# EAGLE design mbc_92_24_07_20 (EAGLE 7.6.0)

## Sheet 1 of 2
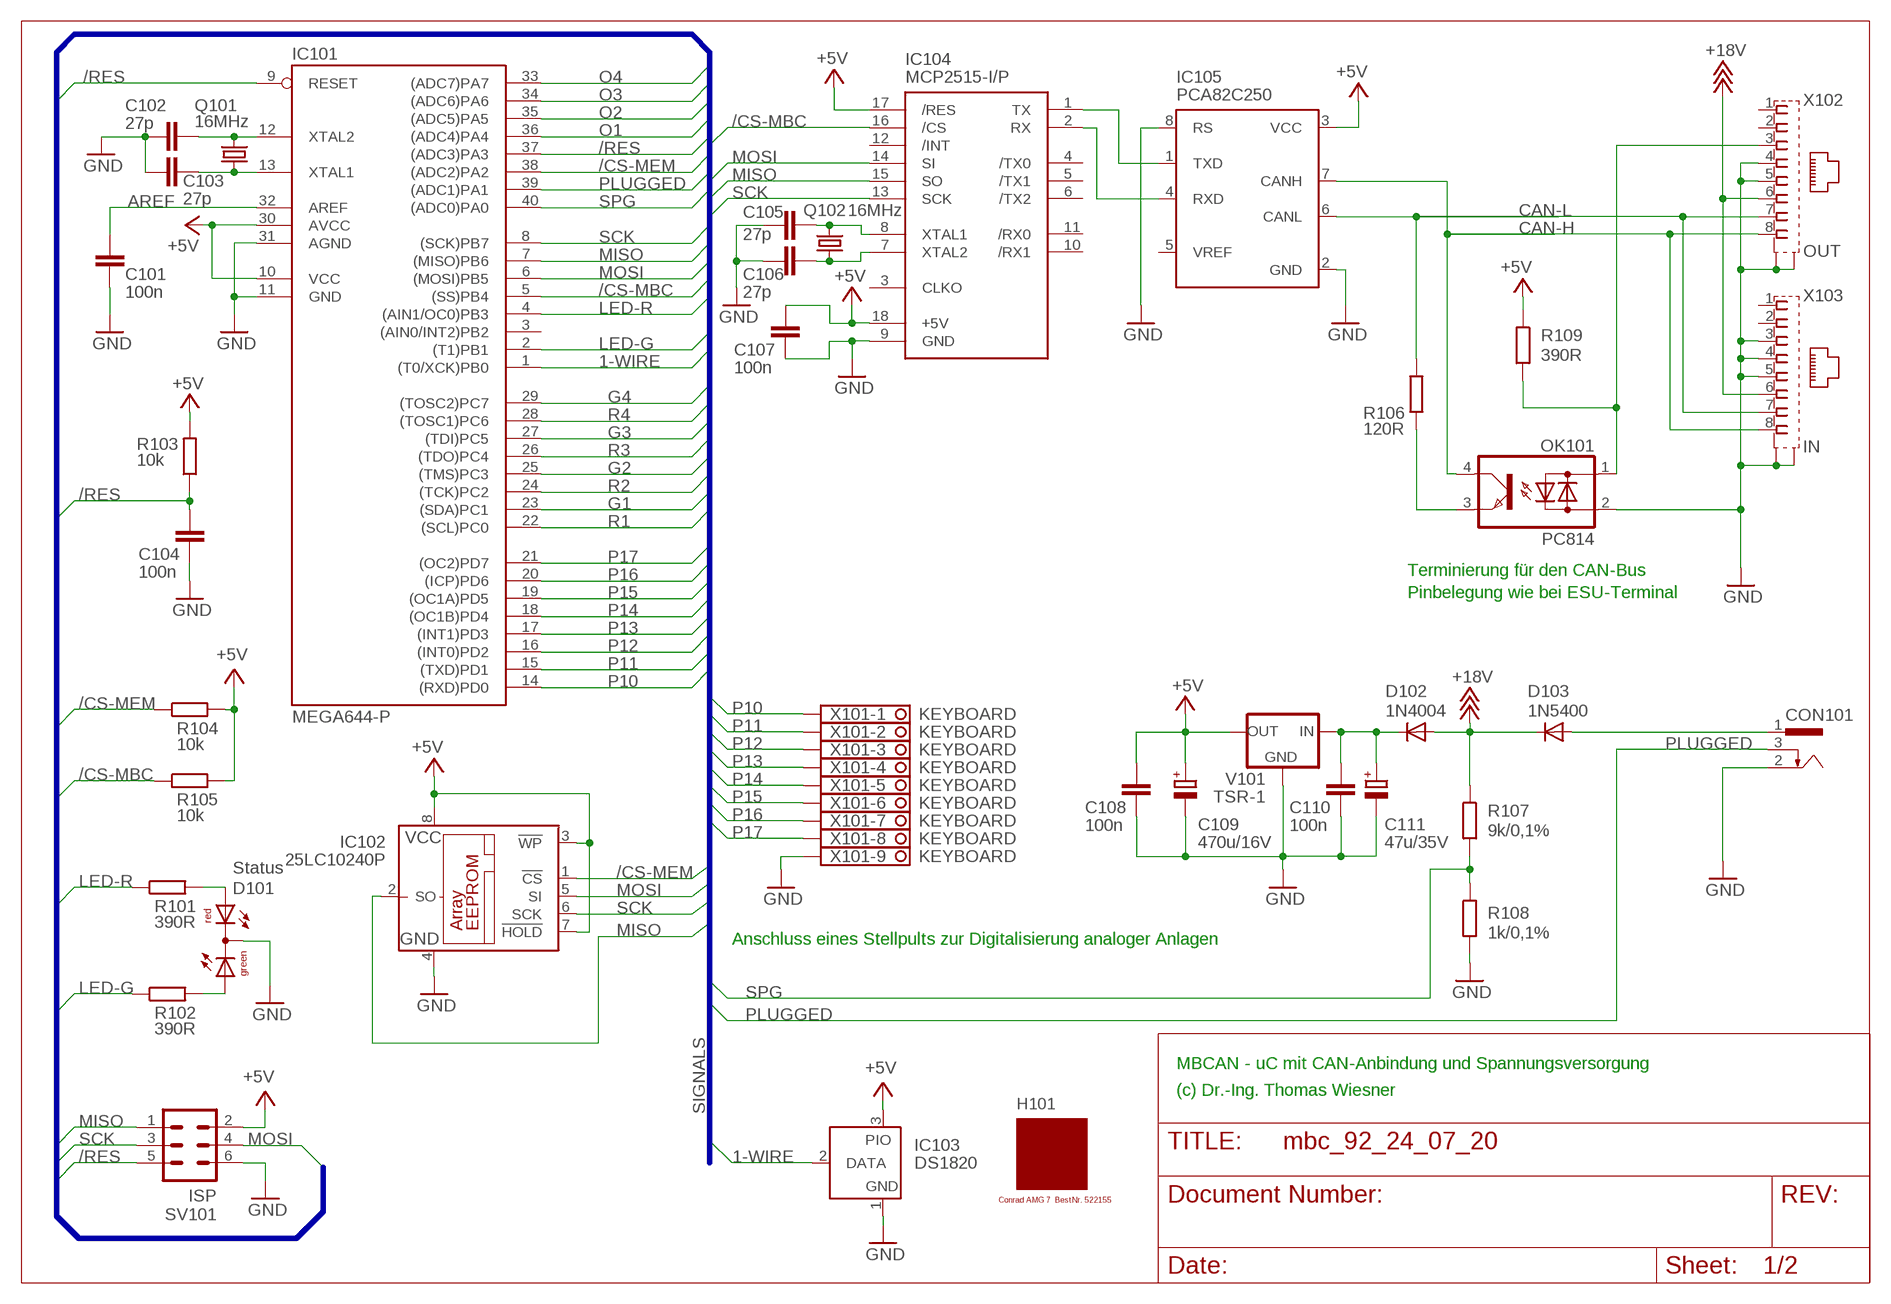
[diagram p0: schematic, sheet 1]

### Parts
C101  100n  C-EU025-025X050  [C025-025X050]
C102  27p  C-EU025-025X050  [C025-025X050]
C103  27p  C-EU025-025X050  [C025-025X050]
C104  100n  C-EU025-025X050  [C025-025X050]
C105  27p  C-EU025-025X050  [C025-025X050]
C106  27p  C-EU025-025X050  [C025-025X050]
C107  100n  C-EU025-025X050  [C025-025X050]
C108  100n  C-EU025-025X050  [C025-025X050]
C109  470u/16V  CPOL-EUE3.5-8  [E3,5-8]
C110  100n  C-EU025-025X050  [C025-025X050]
C111  47u/35V  CPOL-EUE2.5-7  [E2,5-7]
CON101  POWER-JACK  [POWER-JACK]
D101  Status  DUOLED5MM  [DUOLED5MM]
D102  1N4004  [DO41-10]
D103  1N5400  [DO201-15]
H101  MODULGEHÄUSE-AMG-7  [MODULGEHÄUSE-1]
IC101  MEGA644-P  MEGA323-P  [DIL40]
IC102  25LC10240P  25LC040P  [DIL8]
IC103  DS1820  DS2405  [TO92-]
IC104  MCP2515-I/P  MCP2510-I/P  [DIL18]
IC105  PCA82C250  [DIL08]
OK101  PC814  [DIL04]
Q101  16MHz  CRYSTALHC49U70  [HC49U70]
Q102  16MHz  CRYSTALHC49U70  [HC49U70]
R101  390R  R-EU_0207/10  [0207/10]
R102  390R  R-EU_0207/10  [0207/10]
R103  10k  R-EU_0207/10  [0207/10]
R104  10k  R-EU_0207/10  [0207/10]
R105  10k  R-EU_0207/10  [0207/10]
R106  120R  R-EU_0207/10  [0207/10]
R107  9k/0,1%  R-EU_0207/10  [0207/10]
R108  1k/0,1%  R-EU_0207/10  [0207/10]
R109  390R  R-EU_0207/10  [0207/10]
SV101  ISP  ML6  [ML6]
V101  TSR-1  [TRACO-TSR-1]
X101  KEYBOARD  1751316  [1751316]
X102  OUT  0446200002  [0446200002]
X103  IN  0446200002  [0446200002]

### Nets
1-WIRE: IC101.1((T0/XCK)PB0) IC103.2(DATA)
+5V: C107.1 C108.1 C109.+ IC101.10(VCC) IC101.30(AVCC) IC102.3(!WP) IC102.7(!HOLD) IC102.8(VCC) IC103.3(PIO) IC104.17(/RES) IC104.18(+5V) IC105.3(VCC) R103.2 R104.2 R105.2 R109.1 SV101.2 V101.OUT ; also sheet 2
+18V: D102.A D103.C R107.1 X102.6 X103.6
/CS-MBC: IC101.5((SS)PB4) IC104.16(/CS) R105.1
/CS-MEM: IC101.38((ADC2)PA2) IC102.1(!CS) R104.1
/RES: C104.1 IC101.9(RESET) IC101.37((ADC3)PA3) R103.1 SV101.5
AREF: C101.1 IC101.32(AREF)
CAN-H: IC105.7(CANH) OK101.4(C) X102.8 X103.8
CAN-L: IC105.6(CANL) R106.2 X102.7 X103.7
G1: IC101.23((SDA)PC1) ; also sheet 2
G2: IC101.25((TMS)PC3) ; also sheet 2
G3: IC101.27((TDI)PC5) ; also sheet 2
G4: IC101.29((TOSC2)PC7) ; also sheet 2
GND: C101.2 C102.1 C103.1 C104.2 C105.1 C106.1 C107.2 C108.2 C109.- C110.2 C111.- CON101.2 D101.K(C) IC101.11(GND) IC101.31(AGND) IC102.4(GND) IC103.1(GND) IC104.9(GND) IC105.2(GND) IC105.8(RS) OK101.2(AC2) R108.2 SV101.6 V101.GND X101.9 X102.4 X102.5 X102.S@1(S1) X102.S@2(S2) X103.3 X103.4 X103.5 X103.S@1(S1) X103.S@2(S2) ; also sheet 2
LED-G: IC101.2((T1)PB1) R102.1
LED-R: IC101.4((AIN1/OC0)PB3) R101.1
MISO: IC101.7((MISO)PB6) IC102.2(SO) IC104.15(SO) SV101.1
MOSI: IC101.6((MOSI)PB5) IC102.5(SI) IC104.14(SI) SV101.4
N$1: IC104.1(TX) IC105.1(TXD)
N$2: IC104.2(RX) IC105.4(RXD)
N$3: OK101.3(E) R106.1
N$4: OK101.1(AC1) R109.2 X102.3
N$6: C110.1 C111.+ D102.C V101.IN
N$9: D101.AR R101.2
N$13: D101.AG R102.2
N$40: C102.2 IC101.12(XTAL2) Q101.2
N$41: C103.2 IC101.13(XTAL1) Q101.1
N$42: C105.2 IC104.8(XTAL1) Q102.2
N$43: C106.2 IC104.7(XTAL2) Q102.1
O1: IC101.36((ADC4)PA4) ; also sheet 2
O2: IC101.35((ADC5)PA5) ; also sheet 2
O3: IC101.34((ADC6)PA6) ; also sheet 2
O4: IC101.33((ADC7)PA7) ; also sheet 2
P10: IC101.14((RXD)PD0) X101.1
P11: IC101.15((TXD)PD1) X101.2
P12: IC101.16((INT0)PD2) X101.3
P13: IC101.17((INT1)PD3) X101.4
P14: IC101.18((OC1B)PD4) X101.5
P15: IC101.19((OC1A)PD5) X101.6
P16: IC101.20((ICP)PD6) X101.7
P17: IC101.21((OC2)PD7) X101.8
PLUGGED: CON101.3 IC101.39((ADC1)PA1)
R1: IC101.22((SCL)PC0) ; also sheet 2
R2: IC101.24((TCK)PC2) ; also sheet 2
R3: IC101.26((TDO)PC4) ; also sheet 2
R4: IC101.28((TOSC1)PC6) ; also sheet 2
SCK: IC101.8((SCK)PB7) IC102.6(SCK) IC104.13(SCK) SV101.3
SPG: IC101.40((ADC0)PA0) R107.2 R108.1
V-NETZTEIL1: CON101.1 D103.A
Unconnected: IC101.3((AIN0/INT2)PB2) IC104.3(CLKO) IC104.4(/TX0) IC104.5(/TX1) IC104.6(/TX2) IC104.10(/RX1) IC104.11(/RX0) IC104.12(/INT) IC105.5(VREF) X102.1 X102.2 X103.1 X103.2

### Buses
SIGNALS

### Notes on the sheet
- Terminierung für den CAN-Bus
- Pinbelegung wie bei ESU-Terminal
- Anschluss eines Stellpults zur Digitalisierung analoger Anlagen
- MBCAN - uC mit CAN-Anbindung und Spannungsversorgung
- (c) Dr.-Ing. Thomas Wiesner

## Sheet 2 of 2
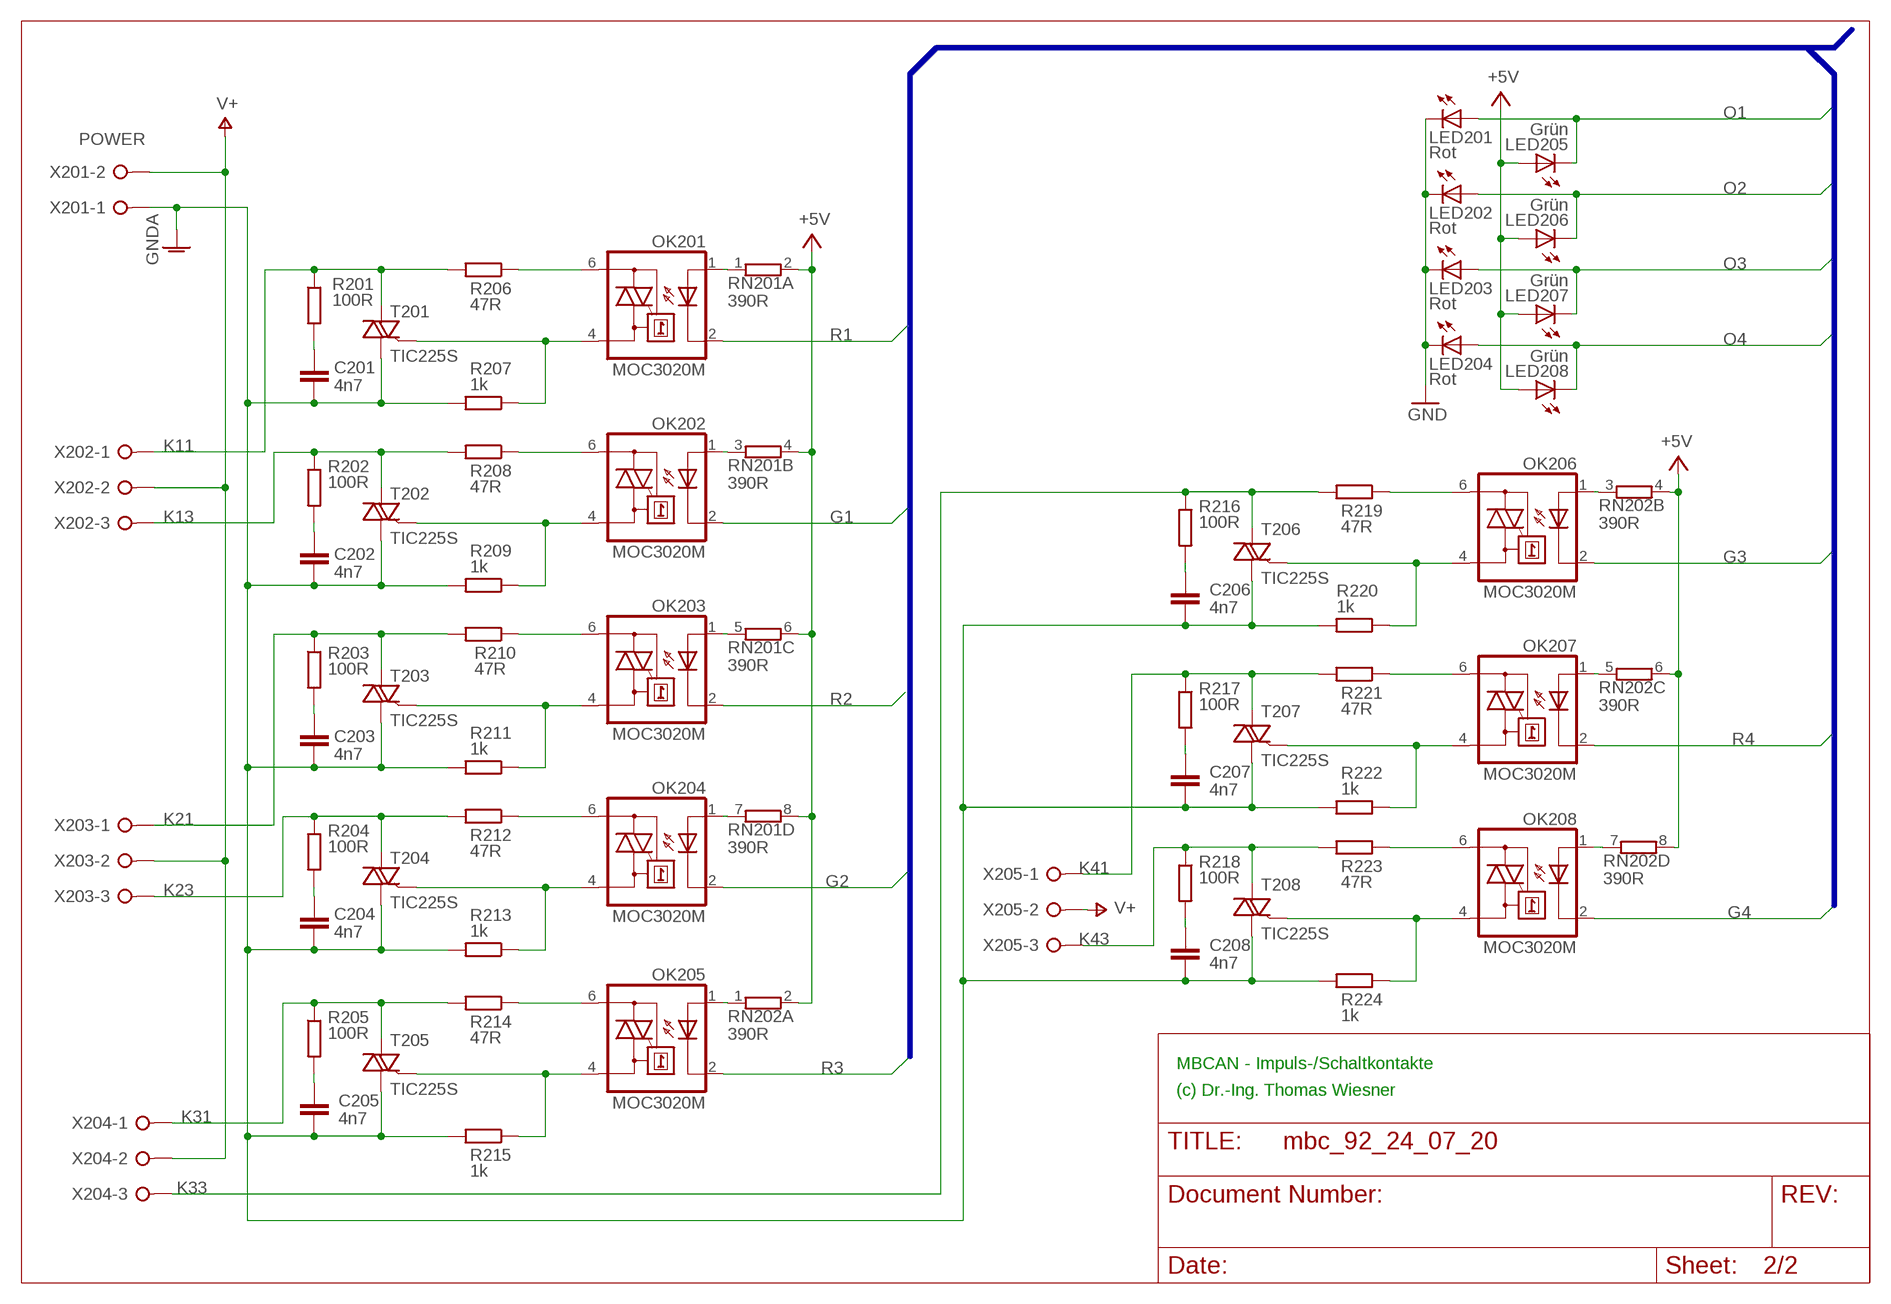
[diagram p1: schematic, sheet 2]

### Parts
C201  4n7  C-EU025-025X050  [C025-025X050]
C202  4n7  C-EU025-025X050  [C025-025X050]
C203  4n7  C-EU025-025X050  [C025-025X050]
C204  4n7  C-EU025-025X050  [C025-025X050]
C205  4n7  C-EU025-025X050  [C025-025X050]
C206  4n7  C-EU025-025X050  [C025-025X050]
C207  4n7  C-EU025-025X050  [C025-025X050]
C208  4n7  C-EU025-025X050  [C025-025X050]
LED201  Rot  LED3MM  [LED3MM]
LED202  Rot  LED3MM  [LED3MM]
LED203  Rot  LED3MM  [LED3MM]
LED204  Rot  LED3MM  [LED3MM]
LED205  Grün  LED3MM  [LED3MM]
LED206  Grün  LED3MM  [LED3MM]
LED207  Grün  LED3MM  [LED3MM]
LED208  Grün  LED3MM  [LED3MM]
OK201  MOC3020M  [DIL06]
OK202  MOC3020M  [DIL06]
OK203  MOC3020M  [DIL06]
OK204  MOC3020M  [DIL06]
OK205  MOC3020M  [DIL06]
OK206  MOC3020M  [DIL06]
OK207  MOC3020M  [DIL06]
OK208  MOC3020M  [DIL06]
R201  100R  R-EU_0207/10  [0207/10]
R202  100R  R-EU_0207/10  [0207/10]
R203  100R  R-EU_0207/10  [0207/10]
R204  100R  R-EU_0207/10  [0207/10]
R205  100R  R-EU_0207/10  [0207/10]
R206  47R  R-EU_0207/10  [0207/10]
R207  1k  R-EU_0207/10  [0207/10]
R208  47R  R-EU_0207/10  [0207/10]
R209  1k  R-EU_0207/10  [0207/10]
R210  47R  R-EU_0207/10  [0207/10]
R211  1k  R-EU_0207/10  [0207/10]
R212  47R  R-EU_0207/10  [0207/10]
R213  1k  R-EU_0207/10  [0207/10]
R214  47R  R-EU_0207/10  [0207/10]
R215  1k  R-EU_0207/10  [0207/10]
R216  100R  R-EU_0207/10  [0207/10]
R217  100R  R-EU_0207/10  [0207/10]
R218  100R  R-EU_0207/10  [0207/10]
R219  47R  R-EU_0207/10  [0207/10]
R220  1k  R-EU_0207/10  [0207/10]
R221  47R  R-EU_0207/10  [0207/10]
R222  1k  R-EU_0207/10  [0207/10]
R223  47R  R-EU_0207/10  [0207/10]
R224  1k  R-EU_0207/10  [0207/10]
RN201  390R  E4R  [SIL8]
RN202  390R  E4R  [SIL8]
T201  TIC225S  [TO220DS]
T202  TIC225S  [TO220DS]
T203  TIC225S  [TO220DS]
T204  TIC225S  [TO220DS]
T205  TIC225S  [TO220DS]
T206  TIC225S  [TO220DS]
T207  TIC225S  [TO220DS]
T208  TIC225S  [TO220DS]
X201  POWER  W237-02P  [W237-132]
X202  W237-03P  [W237-133]
X203  W237-03P  [W237-133]
X204  W237-03P  [W237-133]
X205  W237-03P  [W237-133]

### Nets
+5V: LED205.A LED206.A LED207.A LED208.A RN201.2 RN201.4 RN201.6 RN201.8 RN202.2 RN202.4 RN202.6 RN202.8 ; also sheet 1
G1: OK202.2(C) ; also sheet 1
G2: OK204.2(C) ; also sheet 1
G3: OK206.2(C) ; also sheet 1
G4: OK208.2(C) ; also sheet 1
GND: LED201.K(C) LED202.K(C) LED203.K(C) LED204.K(C) ; also sheet 1
GNDA: C201.2 C202.2 C203.2 C204.2 C205.2 C206.2 C207.2 C208.2 R207.2 R209.2 R211.2 R213.2 R215.2 R220.2 R222.2 R224.2 T201.A1 T202.A1 T203.A1 T204.A1 T205.A1 T206.A1 T207.A1 T208.A1 X201.1
K11: R201.1 R206.2 T201.A2 X202.1
K13: R202.1 R208.2 T202.A2 X202.3
K21: R203.1 R210.2 T203.A2 X203.1
K23: R204.1 R212.2 T204.A2 X203.3
K31: R205.1 R214.2 T205.A2 X204.1
K33: R216.1 R219.2 T206.A2 X204.3
K41: R217.1 R221.2 T207.A2 X205.1
K43: R218.1 R223.2 T208.A2 X205.3
N$5: OK206.1(A) RN202.3
N$7: OK201.1(A) RN201.1
N$8: OK206.4(A1) R220.1 T206.G
N$10: OK201.4(A1) R207.1 T201.G
N$11: OK201.6(A2) R206.1
N$12: OK202.1(A) RN201.3
N$14: OK206.6(A2) R219.1
N$15: C201.1 R201.2
N$16: C206.1 R216.2
N$17: OK202.4(A1) R209.1 T202.G
N$18: OK202.6(A2) R208.1
N$19: OK207.1(A) RN202.5
N$20: C202.1 R202.2
N$21: OK203.1(A) RN201.5
N$22: OK207.4(A1) R222.1 T207.G
N$23: OK203.4(A1) R211.1 T203.G
N$24: OK203.6(A2) R210.1
N$25: OK207.6(A2) R221.1
N$26: C203.1 R203.2
N$27: OK204.1(A) RN201.7
N$28: C207.1 R217.2
N$29: OK204.4(A1) R213.1 T204.G
N$30: OK204.6(A2) R212.1
N$31: OK208.1(A) RN202.7
N$32: C204.1 R204.2
N$33: OK205.1(A) RN202.1
N$34: OK208.4(A1) R224.1 T208.G
N$35: OK205.4(A1) R215.1 T205.G
N$36: OK205.6(A2) R214.1
N$37: OK208.6(A2) R223.1
N$38: C205.1 R205.2
N$39: C208.1 R218.2
O1: LED201.A LED205.K(C) ; also sheet 1
O2: LED202.A LED206.K(C) ; also sheet 1
O3: LED203.A LED207.K(C) ; also sheet 1
O4: LED204.A LED208.K(C) ; also sheet 1
R1: OK201.2(C) ; also sheet 1
R2: OK203.2(C) ; also sheet 1
R3: OK205.2(C) ; also sheet 1
R4: OK207.2(C) ; also sheet 1
V+: X201.2 X202.2 X203.2 X204.2 X205.2

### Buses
B$1

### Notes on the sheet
- MBCAN - Impuls-/Schaltkontakte
- (c) Dr.-Ing. Thomas Wiesner

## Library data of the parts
C101-C108 C110 = rcl:C-EU: CAPACITOR, European symbol
C109 C111 = rcl:CPOL-EU: POLARIZED CAPACITOR, European symbol
C201-C208 = resistor:C-EU: CAPACITOR, European symbol
CON101 = mbc:POWER-JACK: Power-Stecker für 2,5 mm Hohlbuchse
D101 = led:DUOLED5MM: DUO LED 2 colors, 5 mm, round
D102 = diode:1N4004: DIODE
D103 = diode:1N5400: DIODE
H101 = mbc:MODULGEHÄUSE-AMG-7: Gehäuse
IC101 = atmel:MEGA323-P: MICROCONTROLLER 32 Kbytes FLASH 2 Kbytes SRAM 1 Kbytes EEPROM USART 8-channel 10 bit ADC Source: avr.lbr; OC_FARNELL: unknown; OC_NEWARK: unknown
IC102 = microchip:25*: Serial EEPROM 4K/ 8K , SPI bus; MF: MICROCHIP; MPN: 25LC040/P; OC_FARNELL: 9758100; OC_NEWARK: 96K4091
IC103 = maxim:DS2405: Addressable Switch DALLAS Semiconductor; MF: DALLAS SEMICONDUCTOR; MPN: DS2405; OC_FARNELL: 1188025; OC_NEWARK: 06F4645
IC104 = mbc:MCP2510: BASIC-CAN 2.0a Controller Stand-alone CAN controller von Microchip
IC105 = micro-philips:PCA82C250: CAN CONTROLLER INTERFACE; OC_FARNELL: 3692358; OC_NEWARK: unknown
LED201-LED208 = led:LED: LED
OK101 = optocoupler:PC814: SHARP OPTO COUPLER; OC_FARNELL: 9707662; OC_NEWARK: unknown
OK201-OK208 = optocoupler:MOC30*M: RANDOM-PHASE OPTOISOLATORS TRIAC DRIVER OUTPUT Source: http://www.fairchildsemi.com MOC3020-M.pdf; MF: FAIRCHILD SEMICONDUCTOR; MPN: MOC3020-M; OC_FARNELL: 1505425; OC_NEWARK: 72K8895
Q101 Q102 = crystal:CRYSTAL: CRYSTAL; OC_FARNELL: unknown; OC_NEWARK: unknown
R101-R109 R201-R224 = resistor:R-EU_: RESISTOR, European symbol
RN201 RN202 = resistor-sil:E4R: SIL RESISTOR; OC_FARNELL: unknown; OC_NEWARK: unknown
SV101 = con-ml:ML6: HARTING; OC_FARNELL: unknown; OC_NEWARK: unknown
T201-T208 = triac:TIC225S: TRIAC
V101 = mbc:TSR-1: Spannungsregler Hersteller: TRACO Typ: TSR-1 5V: TSR 1-2450 Spg: 5V Strom: 1A Reichelt TSR 1-2450
X101 = con-phoenix-350:1751316: MKDS 1/ 9-3,5 Printklemme Nennstrom: 10 A Bemessungsspannung: 160 V Raster: 3,5 mm Polzahl: 9 Montageart: Löten Anschlussart: Schraubanschluss Anschlussrichtung vom Leiter zur Platine: 0° Source: http://eshop.phoenixcontact.com .. 1751316.pdf; OC_FARNELL: unknown; OC_NEWARK: unknown
X102 X103 = mbc:0446200002: RJ-45 INVERTED MODULAR JACK ASSEMBLY WITH RJ-11 KEEPOUT FEATURE Source: Data sheet MOLEX 0446200002 BUCHSE, RJ45, GESCHIRMT Source: Farnell; MF: MOLEX; MPN: 0446200002; OC_FARNELL: 9251910
X201 = con-wago-508:W237-02P: WAGO SREW CLAMP; OC_FARNELL: unknown; OC_NEWARK: unknown
X202-X205 = con-wago-508:W237-03P: WAGO SREW CLAMP; OC_FARNELL: unknown; OC_NEWARK: unknown

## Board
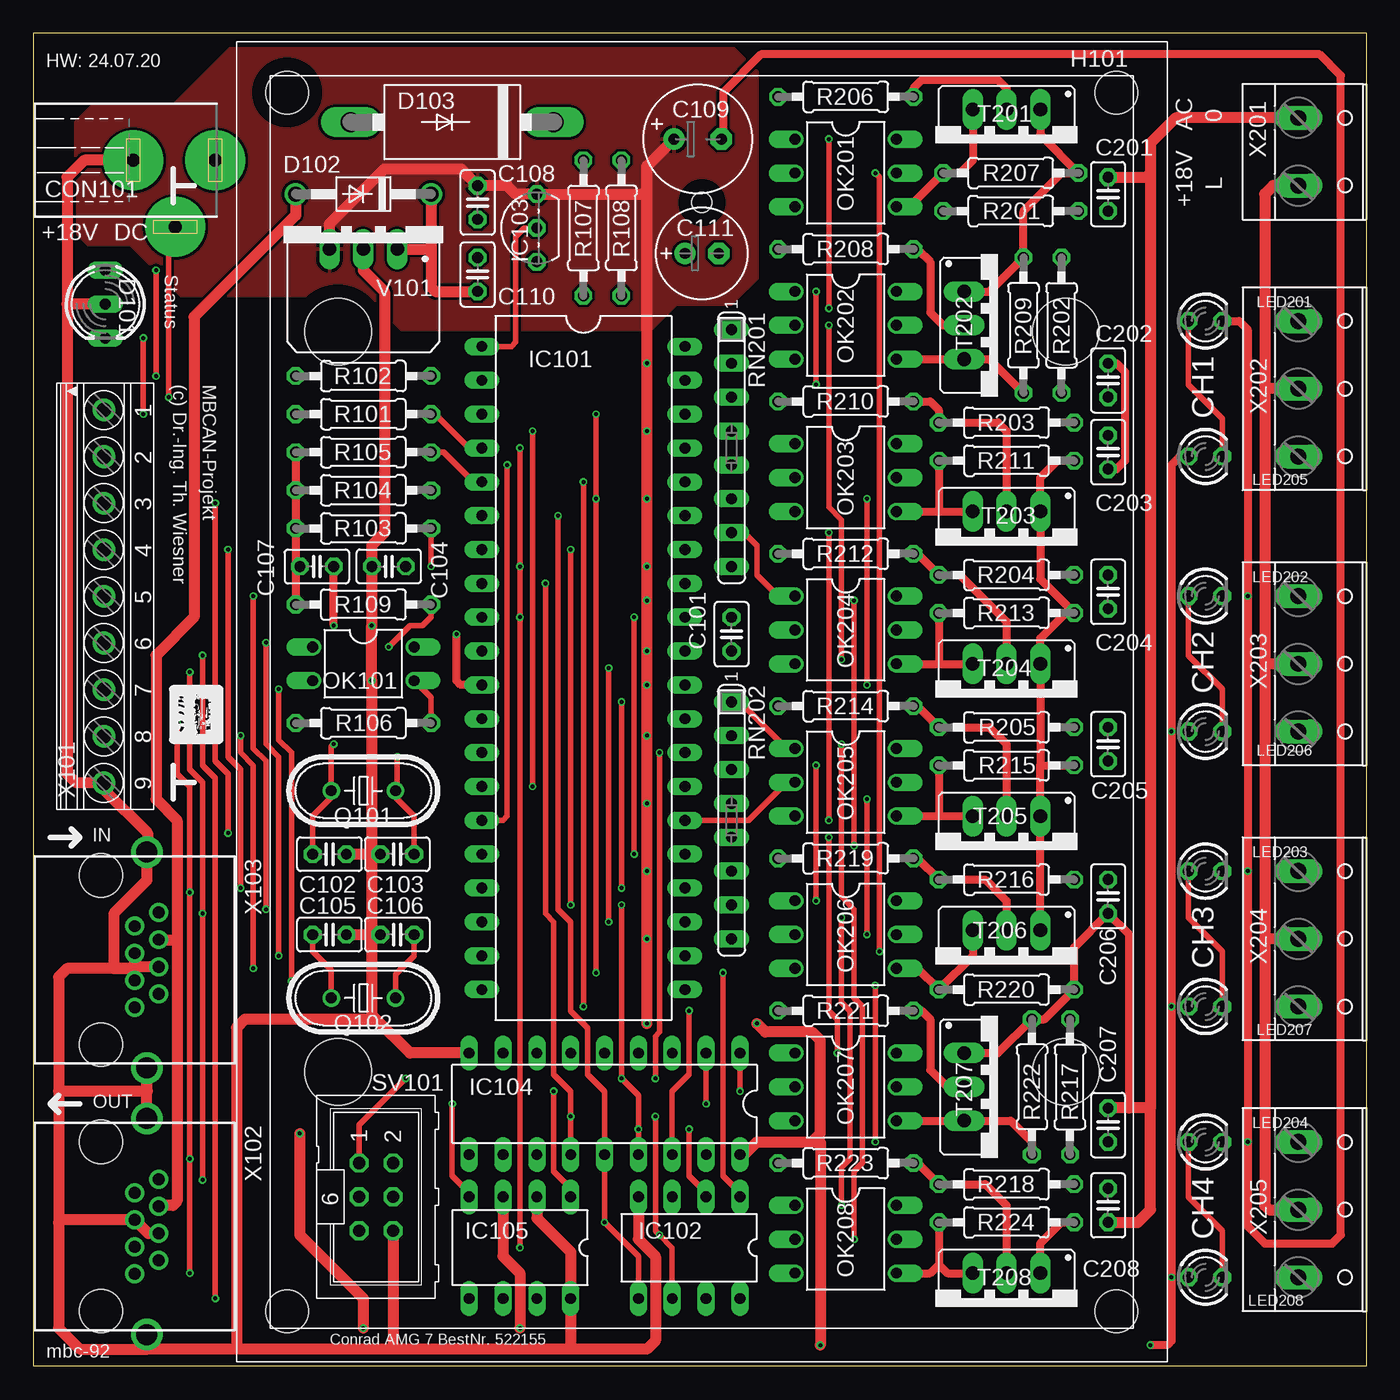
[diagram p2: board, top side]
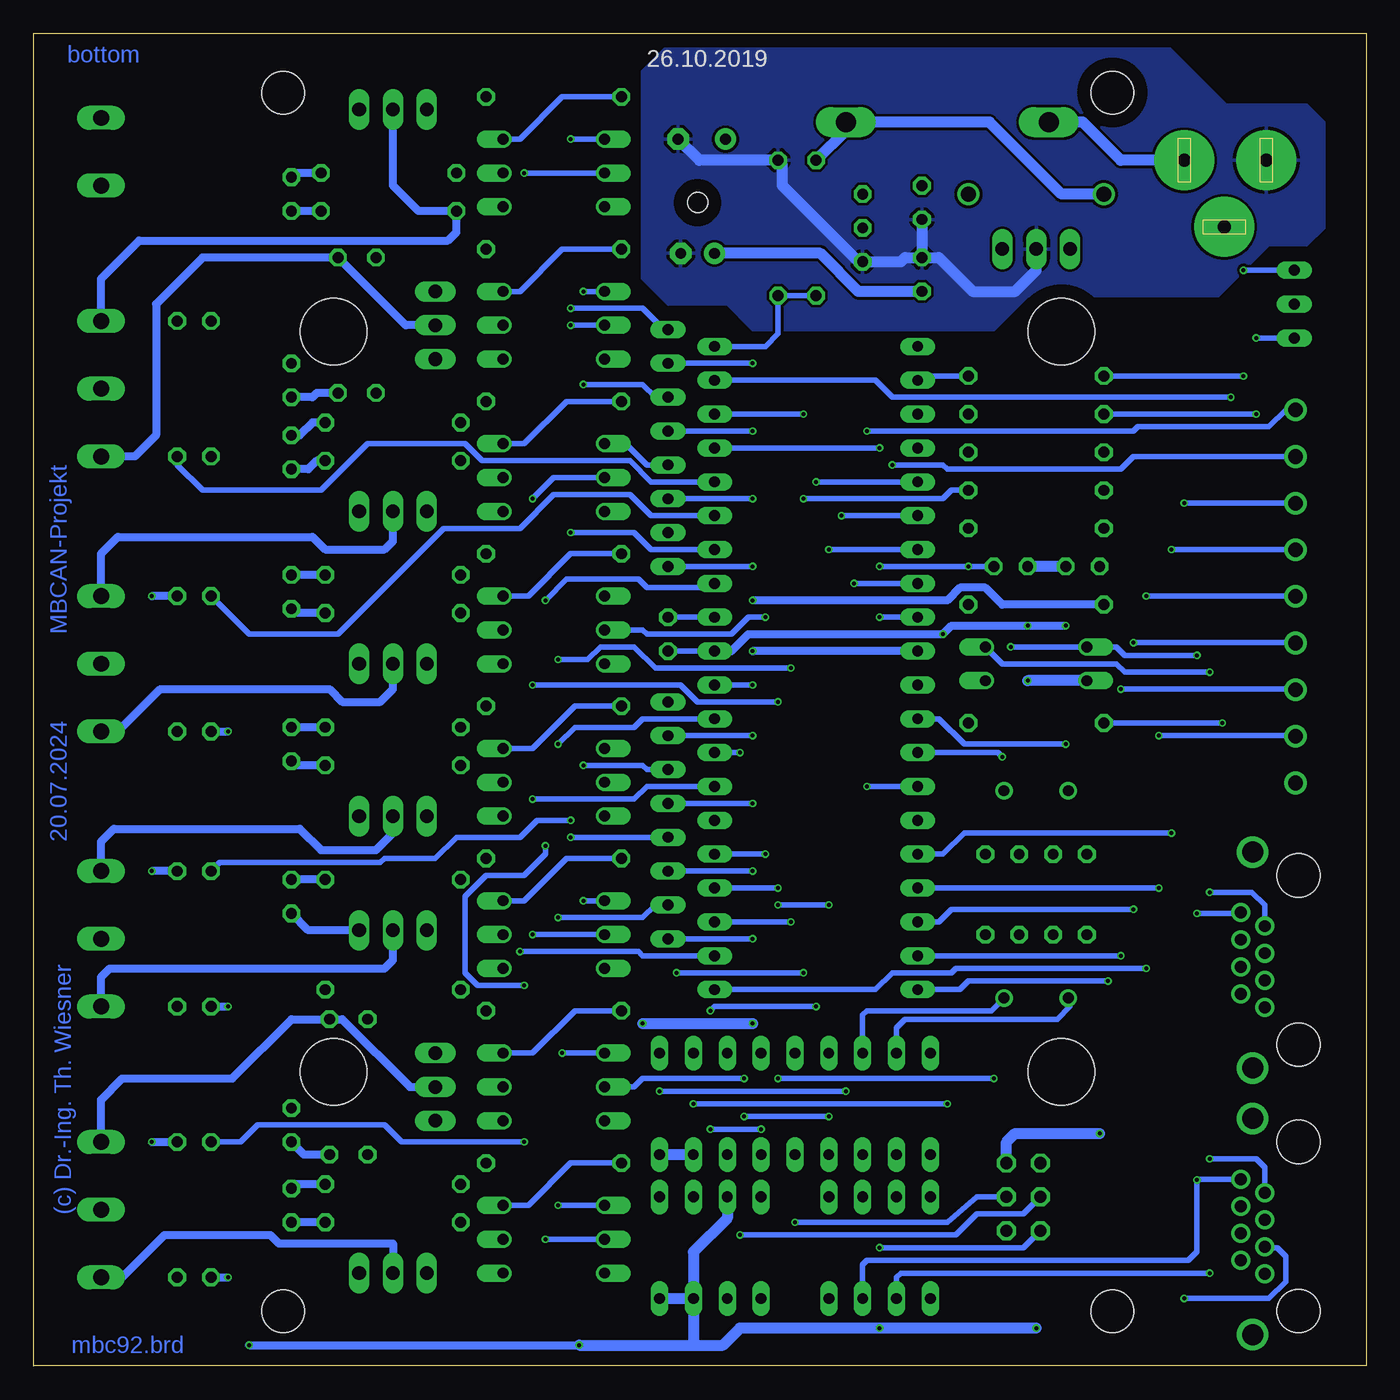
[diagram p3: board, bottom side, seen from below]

Size 100.01 x 100.01 mm. Coordinates in mm from the lower left corner, seen from the top.
Outline: 100,0.02 0,0.02 0,100.01 100,100.01
Outline: 100.01,100.01 100.01,0
Copper layers (1*16): Top 0.035mm / dielectric 1.5mm / Bottom 0.035mm
Design rules "default *": minimum track width 10mil, minimum drill 0.3mm, track to track 8mil, track to pad 8mil, pad to pad 8mil, via to via 8mil, smd to smd 8mil, copper to edge 40mil, drill to drill 8mil, minimum pad ring 10mil, minimum via ring 0.125mm, stop-mask expansion 4mil, vias tented up to drill 0mil, thermal gap 10mil

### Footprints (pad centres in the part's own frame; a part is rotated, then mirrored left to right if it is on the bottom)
C025-025X050 = drill 0.813 octagon: 1 -1.27,0; 2 1.27,0
E3,5-8 = drill 0.813 pad 1.6: + -1.778,0 | drill 0.813 pad 1.6 octagon: - 1.778,0
E2,5-7 = drill 0.813 pad 1.6: + -1.27,0 | drill 0.813 pad 1.6 octagon: - 1.27,0
POWER-JACK = drill 1 pad 4.5: 1 0,6.03; 2 0,-0.12; 3 5,3.03
DUOLED5MM = drill 0.813 long: AG -2.54,0; AR 2.54,0; K 0,0
DO41-10 = drill 1.118: A 5.08,0; C -5.08,0
DO201-15 = drill 1.499 long: A 7.62,0; C -7.62,0
MODULGEHÄUSE-1 = hole 3.2: -45.72,-31.115; -45.72,31.115; 45.72,31.115; 45.72,-31.115 | hole 5: -27.781,-27.305; 27.781,-27.305; -27.781,27.305; 27.781,27.305 | hole 1.5: -37.465,0
DIL40 = drill 0.813 long: 1 -24.13,-7.62; 2 -21.59,-7.62; 3 -19.05,-7.62; 4 -16.51,-7.62; 5 -13.97,-7.62; 6 -11.43,-7.62; 7 -8.89,-7.62; 8 -6.35,-7.62; 9 -3.81,-7.62; 10 -1.27,-7.62; 11 1.27,-7.62; 12 3.81,-7.62; 13 6.35,-7.62; 14 8.89,-7.62; 15 11.43,-7.62; 16 13.97,-7.62; 17 16.51,-7.62; 18 19.05,-7.62; 19 21.59,-7.62; 20 24.13,-7.62; 21 24.13,7.62; 22 21.59,7.62; 23 19.05,7.62; 24 16.51,7.62; 25 13.97,7.62; 26 11.43,7.62; 27 8.89,7.62; 28 6.35,7.62; 29 3.81,7.62; 30 1.27,7.62; 31 -1.27,7.62; 32 -3.81,7.62; 33 -6.35,7.62; 34 -8.89,7.62; 35 -11.43,7.62; 36 -13.97,7.62; 37 -16.51,7.62; 38 -19.05,7.62; 39 -21.59,7.62; 40 -24.13,7.62
DIL8 = drill 0.813 long: 1 -3.81,-3.81; 2 -1.27,-3.81; 3 1.27,-3.81; 4 3.81,-3.81; 5 3.81,3.81; 6 1.27,3.81; 7 -1.27,3.81; 8 -3.81,3.81
TO92- = drill 0.813 octagon: 1 -2.54,0; 2 0,0; 3 2.54,0
DIL18 = drill 0.813 long: 1 -10.16,-3.81; 2 -7.62,-3.81; 3 -5.08,-3.81; 4 -2.54,-3.81 | drill 0.8 long: 5 0,-3.81; 6 2.54,-3.81; 7 5.08,-3.81; 8 7.62,-3.81; 9 10.16,-3.81; 10 10.16,3.81; 11 7.62,3.81; 12 5.08,3.81; 13 2.54,3.81; 14 0,3.81; 15 -2.54,3.81; 16 -5.08,3.81; 17 -7.62,3.81; 18 -10.16,3.81
DIL08 = drill 0.813 long: 1 -3.81,-3.81; 2 -1.27,-3.81; 3 1.27,-3.81; 4 3.81,-3.81; 5 3.81,3.81; 6 1.27,3.81; 7 -1.27,3.81; 8 -3.81,3.81
LED3MM = drill 0.813 octagon: A -1.27,0; K 1.27,0
DIL04 = drill 0.813 offset: 1 -1.27,-3.81; 2 1.27,-3.81; 3 1.27,3.81; 4 -1.27,3.81
DIL06 = drill 0.813 offset: 1 -2.54,-3.81; 2 0,-3.81; 3 2.54,-3.81; 4 2.54,3.81; 5 0,3.81; 6 -2.54,3.81
HC49U70 = drill 0.813: 1 -2.413,0; 2 2.413,0
0207/10 = drill 0.813 octagon: 1 -5.08,0; 2 5.08,0
SIL8 = drill 0.813 long: 1 -8.89,0; 2 -6.35,0; 3 -3.81,0; 4 -1.27,0; 5 1.27,0; 6 3.81,0; 7 6.35,0; 8 8.89,0
ML6 = drill 0.914 octagon: 1 -2.54,-1.27; 2 -2.54,1.27; 3 0,-1.27; 4 0,1.27; 5 2.54,-1.27; 6 2.54,1.27
TO220DS = drill 1.016 long: A1 -2.54,-2.54; A2 0,-2.54; G 2.54,-2.54
TRACO-TSR-1 = drill 1.016 long: GND 0,2.54; IN -2.54,2.54; OUT 2.54,2.54
1751316 = drill 1.1 pad 1.7: 1 -13.973,-0.1; 2 -10.473,-0.1; 3 -6.973,-0.1; 4 -3.473,-0.1; 5 0.028,-0.1; 6 3.527,-0.1; 7 7.027,-0.1; 8 10.527,-0.1; 9 14.027,-0.1
0446200002 = drill 0.889 pad 1.422: 1 3.556,2.54; 2 2.54,4.318; 3 1.524,2.54; 4 0.508,4.318; 5 -0.508,2.54; 6 -1.524,4.318; 7 -2.54,2.54; 8 -3.556,4.318 | drill 1.575 pad 2.286: S@1 -8.103,3.429; S@2 8.103,3.429 | hole 3.251: 6.35,0; -6.35,0
W237-132 = drill 1.194 long: 1 -2.54,-0.635; 2 2.54,-0.635
W237-133 = drill 1.194 long: 1 -5.08,-0.635; 2 0,-0.635; 3 5.08,-0.635

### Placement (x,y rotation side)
C101  52.39,54.93 270 top
C102  22.23,38.42 180 top
C103  27.3,38.42 0 top
C104  26.67,60.01 180 top
C105  22.23,32.38 180 top
C106  27.3,32.38 0 top
C107  21.27,60.01 0 top
C108  33.34,87.31 270 top
C109  49.85,92.08 0 top
C110  33.34,81.92 90 top
C111  50.16,83.5 0 top
C201  80.64,87.95 90 top
C202  80.64,73.98 90 top
C203  80.64,68.58 270 top
C204  80.64,58.1 270 top
C205  80.64,46.67 270 top
C206  80.64,35.24 270 top
C207  80.64,18.1 90 top
C208  80.64,12.06 270 top
CON101  7.62,90.49 270 top
D101  5.4,79.69 270 top
D102  24.77,87.95 180 top
D103  31.43,93.34 180 top
H101  50.16,49.85 270 top
IC101  41.27,52.39 270 top
IC102  49.21,8.89 180 top
IC103  37.78,85.41 90 top
IC104  42.86,19.68 180 top
IC105  36.51,8.89 180 top
LED201  87.95,78.42 0 top
LED202  87.95,57.78 0 top
LED203  87.95,37.15 0 top
LED204  87.95,16.83 0 top
LED205  87.95,68.26 0 top
LED206  87.95,47.62 0 top
LED207  87.95,26.99 0 top
LED208  87.95,6.67 0 top
OK101  24.77,52.7 270 top
OK201  60.96,89.53 270 top
OK202  60.96,78.11 270 top
OK203  60.96,66.67 270 top
OK204  60.96,55.24 270 top
OK205  60.96,43.81 270 top
OK206  60.96,32.38 270 top
OK207  60.96,20.95 270 top
OK208  60.96,9.53 270 top
Q101  24.77,43.18 180 top
Q102  24.77,27.62 180 top
R101  24.77,71.44 180 top
R102  24.77,74.3 180 top
R103  24.77,62.87 180 top
R104  24.77,65.72 180 top
R105  24.77,68.58 180 top
R106  24.77,48.26 180 top
R107  41.27,85.41 270 top
R108  44.13,85.41 90 top
R109  24.77,57.15 0 top
R201  73.34,86.68 0 top
R202  77.15,78.11 270 top
R203  73.03,70.8 0 top
R204  73.03,59.37 0 top
R205  73.03,47.94 0 top
R206  60.96,95.25 0 top
R207  73.34,89.53 0 top
R208  60.96,83.82 0 top
R209  74.3,78.11 90 top
R210  60.96,72.39 0 top
R211  73.03,67.94 0 top
R212  60.96,60.96 0 top
R213  73.03,56.52 0 top
R214  60.96,49.53 0 top
R215  73.03,45.09 0 top
R216  73.03,36.51 0 top
R217  77.79,20.95 270 top
R218  73.03,13.65 0 top
R219  60.96,38.1 0 top
R220  73.03,28.26 0 top
R221  60.96,26.67 0 top
R222  74.93,20.95 90 top
R223  60.96,15.24 0 top
R224  73.03,10.79 0 top
RN201  52.39,68.9 270 top
RN202  52.39,40.96 270 top
SV101  25.72,12.7 270 top
T201  73.03,91.76 180 top
T202  72.39,78.11 270 top
T203  73.03,61.59 180 top
T204  73.03,50.16 180 top
T205  73.03,38.73 180 top
T206  73.03,30.16 180 top
T207  72.39,20.95 270 top
T208  73.03,4.45 180 top
V101  24.77,86.36 180 top
X101  5.4,57.78 270 top
X102  5.08,10.48 270 top
X103  5.08,30.48 270 top
X201  95.57,91.12 270 top
X202  95.57,73.34 270 top
X203  95.57,52.7 270 top
X204  95.57,32.07 270 top
X205  95.57,11.75 270 top

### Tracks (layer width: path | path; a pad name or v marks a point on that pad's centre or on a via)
1-WIRE
  Top 0.406: IC103.2 36.83,85.41 36.2,84.77 36.2,76.83 35.88,76.52 IC101.1
+5V  (via drill 0.3)
  Top 0.61: R105.2 R104.2 R103.2 19.68,60.33 C107.1 19.68,59.69 R109.1 | LED205.A 86.04,68.26 85.41,67.63 v85.41,47.62 v85.41,26.99 v85.41,6.67 85.41,1.91 85.09,1.59 v83.82,1.59
  Top 0.813: 46.04,88.27 v46.04,75.25 v46.04,70.17 v46.04,65.09 v46.04,60.01 v46.04,57.47 v46.04,53.66 v46.04,51.12 v46.04,47.31 v46.04,42.23 v46.04,37.15 v46.04,32.07 v46.04,25.72 | 46.04,88.27 46.04,90.04 C109.+ | 58.42,16.83 54.29,16.83 53.34,15.88 IC104.18 | 58.42,16.83 59.05,17.46 59.05,24.45 58.42,25.08 54.93,25.08 v54.29,25.72 | v20,17.46 20,9.84 24.77,5.08 v24.77,2.86 | 58.42,16.83 59.05,16.83 v59.05,1.59 | IC105.3 35.24,8.26 36.51,6.99 v36.51,2.86 | 46.04,88.27 45.72,87.95 IC103.3 36.2,87.95 35.56,88.58 C108.1 32.07,89.85 26.35,89.85 22.23,85.72 V101.OUT
  Bottom 0.406: RN202.8 v46.04,32.07 | RN202.6 v46.04,37.15 | RN202.4 v46.04,42.23 | RN202.2 v46.04,47.31 | IC101.30 v46.04,51.12 | RN201.8 v46.04,60.01 | RN201.6 v46.04,65.09 | RN201.4 v46.04,70.17 | RN201.2 v46.04,75.25
  Bottom 0.61: v83.82,1.59 v59.05,1.59 | IC101.10 v46.04,53.66 | R109.1 27.3,57.15 28.57,58.42 30.48,58.42 31.43,57.47 v46.04,57.47 | LED208.A v85.41,6.67 | LED207.A v85.41,26.99 | LED206.A v85.41,47.62
  Bottom 0.813: v59.05,1.59 50.48,1.59 | 50.48,1.59 48.26,1.59 46.99,2.86 v36.51,2.86 v24.77,2.86 | v54.29,25.72 v46.04,25.72 | SV101.2 26.99,16.83 26.35,17.46 v20,17.46 | IC102.8 IC102.7 | IC102.7 50.48,1.59 | IC102.3 47.94,11.11 50.48,8.57 IC102.7 | IC104.17 IC104.18
  pour Top: 6.35,94.61 10.48,94.61 14.92,99.06 52.39,99.06 54.29,97.16 54.29,81.6 52.7,80.01 52.39,79.69 48.26,79.69 46.35,77.79 27.62,77.79 25.08,80.33 11.11,80.33 7.3,84.14 4.13,84.14 3.17,85.09 3.17,93.34 4.45,94.61
+18V
  Top 0.813: D102.A 19.68,86.36 12.06,78.74 12.06,56.2 9.21,53.34 9.21,42.55 10.79,40.96 10.79,32.07 | 10.79,32.07 10.79,12.38 10.48,12.06 9.46,12.06 | X103.6 10.73,32 10.79,32.07
  Top 1.016: 9.46,12.06 X102.6
  Bottom 0.813: D102.A 22.86,87.95 28.26,93.34 D103.C | 39.37,93.03 D103.C | D103.C 39.05,92.71 R107.1
/CS-MBC  (via drill 0.3)
  Top 0.406: IC104.16 47.94,20.64 49.21,21.91 v49.21,26.67 | v41.27,26.99 v41.27,66.36 | IC101.5 33.02,66.36 30.8,68.58 R105.1
  Bottom 0.406: v49.21,26.67 48.9,26.99 v41.27,26.99 | v41.27,66.36 IC101.5
/CS-MEM  (via drill 0.3)
  Top 0.406: IC102.1 53.02,13.02 51.75,14.29 v51.75,29.53 | v42.23,29.53 v42.23,65.09 v42.23,71.44
  Bottom 0.406: v51.75,29.53 v42.23,29.53 | v42.23,71.44 IC101.38 | R104.1 31.11,65.72 31.75,65.09 v42.23,65.09
/RES  (via drill 0.3)
  Top 0.406: v36.51,8.89 v36.51,56.2 v36.51,60.01 v36.51,68.9 | R103.1 v29.84,60.01
  Bottom 0.406: SV101.5 25.72,8.89 v36.51,8.89 | v36.51,60.01 v29.84,60.01 C104.1 | IC101.9 v36.51,56.2 | IC101.37 v36.51,68.9
AREF
  Bottom 0.406: IC101.32 C101.1
CAN-H  (via drill 0.3)
  Top 0.406: v11.75,52.07 11.75,44.77 12.7,43.81 v12.7,33.97 v12.7,13.97
  Bottom 0.406: OK101.4 27.3,52.7 18.73,52.7 18.1,52.07 v11.75,52.07 | v12.7,33.97 9.46,33.97 X103.8 | X102.8 12.64,14.03 v12.7,13.97 12.7,8.57 13.34,7.94 37.47,7.94 37.78,7.62 IC105.7
CAN-L  (via drill 0.3)
  Top 0.406: v10.79,48.26 10.79,44.45 11.75,43.5 v11.75,35.56 v11.75,15.56 v11.75,6.99
  Bottom 0.406: X102.7 7.62,14.92 8.26,15.56 v11.75,15.56 | v10.79,48.26 R106.2 | X103.7 7.62,34.61 8.57,35.56 v11.75,35.56 | IC105.6 35.24,6.67 34.92,6.99 v11.75,6.99
G1  (via drill 0.3)
  Top 0.406: v59.69,78.11 59.69,64.45 60.64,63.5 v60.64,53.02 | v43.18,52.39 v43.18,33.34
  Bottom 0.406: OK202.2 v59.69,78.11 | v60.64,53.02 58.42,53.02 57.47,53.98 54.93,53.98 53.34,52.39 v43.18,52.39 | v43.18,33.34 IC101.23
G2  (via drill 0.3)
  Top 0.406: v45.09,56.2 v45.09,38.42
  Bottom 0.406: OK204.2 54.29,55.24 53.98,54.93 47.62,54.93 46.35,56.2 v45.09,56.2 | v45.09,38.42 IC101.25
G3  (via drill 0.3)
  Top 0.406: v62.55,42.55 v62.55,32.38
  Bottom 0.406: IC101.27 53.98,43.5 54.93,42.55 v62.55,42.55 | v62.55,32.38 OK206.2
G4  (via drill 0.3)
  Top 0.406: v60.64,46.67 60.64,35.24 61.59,34.29 61.59,27.62 62.23,26.99 62.23,15.24 61.59,14.61 v61.59,9.53
  Bottom 0.406: IC101.29 54.29,48.58 54.93,47.94 59.37,47.94 v60.64,46.67 | v61.59,9.53 OK208.2
GND  (via drill 0.3)
  Top 0.61: v22.54,55.56 C107.2 | IC101.11 32.07,51.12 31.75,51.44 v31.75,54.93 | LED201.K 90.49,78.42 91.12,77.79 v91.12,57.78 v91.12,37.15 v91.12,16.83 91.12,10.48 92.39,9.21 97.47,9.21 98.11,9.84 98.11,96.84 96.52,98.42 54.61,98.42 51.75,95.57 51.75,92.08 C109.-
  Top 0.813: V101.GND 24.77,82.23 26.35,80.64 26.35,62.55 25.4,61.59 C104.2 v25.4,55.56 v25.4,51.44 25.4,38.42 | 25.4,38.42 25.4,32.38 | 25.4,32.38 25.4,26.35 25.72,26.04 | C105.1 25.4,32.38 | 25.4,32.38 C106.1 | C102.1 25.4,38.42 | C103.1 25.4,38.42 | 7.62,29.84 7.62,30.16 | 7.62,30.16 X103.5 | X103.4 7.81,29.97 7.62,30.16 | 7.62,30.16 7.3,29.84 6.03,29.84 6.03,33.97 8.51,36.45 X103.S@1 8.57,38.65 8.57,40.01 5.3,43.28 X101.9 5.24,43.81 3.17,43.81 2.54,44.45 2.54,79.69 | X103.3 7.62,29.84 | 7.62,29.84 2.54,29.84 1.91,29.21 1.91,20.64 | 1.91,20.64 1.91,10.79 | 1.91,10.79 1.91,2.86 3.49,1.27 8.57,1.27 | 8.57,1.27 8.57,2.31 X102.S@2 | X102.4 8.64,9.97 X102.5 2.1,10.99 1.91,10.79 | X102.S@1 X103.S@2 8.51,20.7 8.57,20.64 1.91,20.64 | 40.32,1.27 IC105.8 40.32,8.57 37.78,11.11 IC105.2 | 40.32,1.27 26.99,1.27 | 26.99,1.27 15.24,1.27 | 15.24,1.27 8.57,1.27 | SV101.6 26.99,1.27 | IC104.9 28.26,23.5 25.72,26.04 | 25.72,26.04 15.88,26.04 15.24,25.4 15.24,1.27 | CON101.2 3.81,90.49 2.54,89.22 2.54,79.69 | D101.K 2.54,79.69 | IC102.4 45.4,9.53 46.67,8.26 46.67,1.91 46.04,1.27 40.32,1.27 | 51.75,92.2 C109.-
  Bottom 0.406: C101.2 IC101.31
  Bottom 0.61: IC101.31 47.62,53.66 46.35,54.93 v31.75,54.93 31.11,55.56 v22.54,55.56 | v91.12,16.83 LED204.K | LED203.K v91.12,37.15 | LED202.K v91.12,57.78
  Bottom 0.813: C107.2 C104.2 | OK101.2 v25.4,51.44 | C109.- 50.04,90.49 R108.2 43.81,90.17 43.81,88.58 38.1,82.87 IC103.1 34.92,82.87 34.61,83.19 C110.2 | C110.2 32.07,83.19 29.53,80.64 26.35,80.64 24.77,82.23 V101.GND | C108.2 C110.2
  pour Bottom: 6.03,94.61 10.48,94.61 15.24,99.38 52.07,99.38 54.29,97.16 54.29,81.6 52.39,79.69 47.94,79.69 46.04,77.79 27.94,77.79 25.4,80.33 11.11,80.33 7.3,84.14 4.45,84.14 3.17,85.41 3.17,93.34 4.45,94.61
GNDA
  Top 0.61: 75.56,45.09 T205.A1 T206.A1 | 75.56,45.09 R215.2 | R211.2 76.83,67.94 75.56,66.67 T203.A1 75.56,59.05 R213.2 77.47,56.52 75.56,54.61 T204.A1 75.56,45.09 | T202.A1 71.75,80.64 R209.2 74.3,86.68 77.15,89.53 R207.2 75.56,92.39 T201.A1 | T207.A1 72.39,23.5 R222.2 75.88,26.04 R220.2 78.11,31.43 C206.2 82.23,32.38 82.23,19.37 | T208.A1 75.56,9.21 77.15,10.79 R224.2 | C202.2 81.28,75.25 81.92,74.61 81.92,67.94 81.28,67.31 C203.2
  Top 0.813: X201.1 85.72,93.66 83.82,91.76 83.82,89.53 | 83.82,89.53 83.82,19.37 | 83.82,19.37 82.23,19.37 C207.2 | C208.2 82.87,10.79 83.82,11.75 83.82,19.37 | C201.2 83.5,89.22 83.82,89.53
  Bottom 0.61: T206.A1 79.38,32.7 C206.2 | R215.2 80.33,45.09 C205.2 | R213.2 80.33,56.52 C204.2 | R211.2 78.74,67.94 79.38,67.31 C203.2 | R207.2 80.33,89.53 C201.2 | R224.2 C208.2
K11
  Top 0.61: R206.2 66.04,95.89 66.67,96.52 72.39,96.52 73.03,95.89 T201.A2
  Bottom 0.61: X202.1 94.93,81.6 92.08,84.45 68.9,84.45 68.26,85.09 R201.1 71.12,86.68 73.03,88.58 T201.A2
K13
  Top 0.61: R208.2 66.36,83.82 67.31,82.87 67.31,79.06 68.26,78.11 T202.A2
  Bottom 0.61: T202.A2 72.07,78.11 R202.1 87.31,83.19 90.81,79.69 90.81,69.85 92.39,68.26 X202.3
K21
  Top 0.61: R210.2 67.31,72.39 67.94,71.75 R203.1 72.39,70.8 73.03,70.17 T203.A2
  Bottom 0.61: X203.1 94.93,60.96 93.66,62.23 79.06,62.23 78.11,61.28 73.66,61.28 73.03,61.91 T203.A2
K23
  Top 0.61: R212.2 66.36,60.96 R204.1 69.53,59.37 73.03,55.88 T204.A2
  Bottom 0.61: X203.3 93.66,47.62 90.49,50.8 77.79,50.8 76.83,49.85 73.98,49.85 73.03,50.8 T204.A2
K31
  Top 0.61: R214.2 66.36,49.53 R205.1 71.75,47.94 73.03,46.67 T205.A2
  Bottom 0.61: X204.1 94.93,39.37 93.98,40.32 80.01,40.32 78.42,38.73 74.3,38.73 73.03,40.01 T205.A2
K33
  Top 0.61: R219.2 66.36,38.1 R216.1 71.44,36.51 73.03,34.92 T206.A2
  Bottom 0.61: X204.3 94.93,29.21 94.3,29.84 73.66,29.84 73.03,30.48 T206.A2
K41
  Top 0.61: R221.2 66.67,26.67 67.31,26.04 67.31,22.23 68.58,20.95 T207.A2
  Bottom 0.61: X205.1 94.93,20 93.34,21.59 85.09,21.59 80.64,26.04 R217.1 76.83,26.04 71.75,20.95 T207.A2
K43
  Top 0.61: T208.A2 73.03,12.06 71.44,13.65 R218.1 66.36,15.24 R223.2
  Bottom 0.61: X205.3 93.34,6.67 90.17,9.84 82.23,9.84 81.6,9.21 73.03,9.21 T208.A2
LED-G
  Bottom 0.406: R102.1 32.7,74.3 33.02,73.98 IC101.2
LED-R
  Top 0.406: R101.1 30.16,71.44 32.7,68.9 IC101.4
MISO  (via drill 0.3)
  Top 0.406: IC104.15 v45.4,17.78 45.4,20.32 v44.13,21.59 v44.13,34.61 | v40.32,34.61 v40.32,61.28 | IC102.2 50.48,13.02 49.21,14.29 v49.21,17.78 | SV101.1 24.45,18.1 v27.94,21.59
  Bottom 0.406: v44.13,34.61 v40.32,34.61 | v40.32,61.28 IC101.7 | v49.21,17.78 v45.4,17.78 | v27.94,21.59 v44.13,21.59
MOSI  (via drill 0.3)
  Top 0.406: v39.37,63.82 39.37,34.29 40.32,33.34 40.32,26.67 41.59,25.4 41.59,21.91 42.86,20.64 IC104.14 v42.86,10.79 45.4,8.26 IC102.5
  Bottom 0.406: v39.37,63.82 IC101.6 | SV101.4 29.21,12.7 31.43,10.79 v42.86,10.79
N$1  (via drill 0.3)
  Top 0.406: IC104.1 v53.02,20.64 | v39.05,20.64 39.05,14.61 40.32,13.34 IC105.1
  Bottom 0.406: v53.02,20.64 v39.05,20.64
N$2  (via drill 0.3)
  Top 0.406: IC105.4 32.7,13.02 31.43,14.29 v31.43,19.68 | v50.48,19.68 IC104.2
  Bottom 0.406: v31.43,19.68 v50.48,19.68
N$3
  Top 0.406: R106.1 29.84,50.16 OK101.3
N$4  (via drill 0.3)
  Top 0.406: R109.2 29.84,56.2 29.21,55.56 28.26,55.56 v26.67,53.98 | v12.7,53.34 12.7,45.09 13.65,44.13 v13.65,5.08
  Bottom 0.406: v26.67,53.98 OK101.1 18.73,53.98 18.1,53.34 v12.7,53.34 | v13.65,5.08 7.3,5.08 6.03,6.35 6.03,8.26 6.67,8.89 7.56,8.89 X102.3
N$5  (via drill 0.3)
  Top 0.406: v58.74,45.09 v58.74,34.92
  Bottom 0.406: RN202.3 53.98,44.77 54.29,45.09 v58.74,45.09 | v58.74,34.92 OK206.1
N$6
  Top 0.813: D102.C 29.84,83.82 | 29.84,83.82 29.84,80.96 30.16,80.64 C110.1 | V101.IN 29.84,83.82
  Bottom 0.813: C110.1 38.1,80.64 40.96,83.5 C111.+
N$7  (via drill 0.3)
  Top 0.406: v59.69,79.38 v59.69,92.08
  Bottom 0.406: RN201.1 52.7,77.79 54.29,79.38 v59.69,79.38 | v59.69,92.08 OK201.1
N$8
  Top 0.61: OK206.4 66.36,29.84 R220.1 70.48,30.8 T206.G
N$9  (via drill 0.3)
  Top 0.406: v8.26,71.44 v8.26,77.15
  Bottom 0.406: R101.2 v8.26,71.44 | v8.26,77.15 D101.AR
N$10
  Top 0.61: T201.G 70.48,90.49 69.53,89.53 R207.1 65.72,87 OK201.4
N$11
  Bottom 0.406: R206.1 60.33,95.25 63.5,92.08 OK201.6
N$12  (via drill 0.3)
  Top 0.406: v58.74,73.66 v58.74,80.64
  Bottom 0.406: RN201.3 53.34,72.71 54.29,73.66 v58.74,73.66 | v58.74,80.64 OK202.1
N$13  (via drill 0.3)
  Top 0.406: v9.21,74.3 v9.21,82.23
  Bottom 0.406: R102.2 v9.21,74.3 | v9.21,82.23 D101.AG
N$14
  Bottom 0.406: R219.1 60.01,38.1 63.18,34.92 OK206.6
N$15
  Bottom 0.61: R201.2 C201.1
N$16
  Bottom 0.61: R216.2 C206.1
N$17
  Top 0.61: OK202.4 T202.G 71.75,75.56 R209.1
N$18
  Bottom 0.406: R208.1 60.33,83.82 63.5,80.64 OK202.6
N$19  (via drill 0.3)
  Top 0.406: v59.69,39.69 59.69,26.67 60.33,26.04 v60.33,23.5
  Bottom 0.406: RN202.5 v59.69,39.69 | v60.33,23.5 OK207.1
N$20
  Bottom 0.61: R202.2 78.74,73.03 79.06,72.71 C202.1
N$21
  Bottom 0.406: RN201.5 53.98,67.63 55.56,69.22 OK203.1
N$22
  Top 0.61: OK207.4 T207.G 73.34,18.41 74.93,16.83 R222.1
N$23
  Top 0.61: OK203.4 67.94,64.14 | 67.94,64.14 T203.G | R211.1 67.94,64.14
N$24
  Bottom 0.406: R210.1 60.01,72.39 63.18,69.22 OK203.6
N$25
  Bottom 0.406: R221.1 59.37,26.67 62.55,23.5 OK207.6
N$26
  Bottom 0.61: R203.2 79.06,70.8 80.01,69.85 C203.1
N$27
  Top 0.406: RN201.7 53.34,62.55 54.29,61.59 54.29,59.37 55.88,57.78 OK204.1
N$28
  Bottom 0.61: R217.2 79.69,15.88 C207.1
N$29
  Top 0.61: OK204.4 67.94,52.7 | 67.94,52.7 T204.G | R213.1 67.94,52.7
N$30
  Bottom 0.406: R212.1 59.69,60.96 62.87,57.78 OK204.6
N$31  (via drill 0.3)
  Top 0.406: v60.64,33.66 60.64,27.3 61.28,26.67 61.28,15.56 60.64,14.92 v60.64,12.06
  Bottom 0.406: RN202.7 53.34,34.61 54.29,33.66 v60.64,33.66 | v60.64,12.06 OK208.1
N$32
  Bottom 0.61: R204.2 C204.1
N$33
  Top 0.406: RN202.1 53.02,49.85 56.52,46.35 OK205.1
N$34
  Top 0.61: R224.1 67.94,7.62 | 67.94,7.62 68.58,6.99 T208.G | OK208.4 67.31,6.99 67.94,7.62
N$35
  Top 0.61: OK205.4 67.94,41.27 | 67.94,41.27 T205.G | R215.1 67.94,41.27
N$36
  Bottom 0.406: R214.1 59.37,49.53 62.55,46.35 OK205.6
N$37
  Bottom 0.406: R223.1 59.69,15.24 62.87,12.06 OK208.6
N$38
  Bottom 0.61: R205.2 C205.1
N$39
  Bottom 0.61: R218.2 80.33,13.65 C208.1
N$40  (via drill 0.3)
  Top 0.406: C102.2 20.95,41.27 22.35,42.67 Q101.2 22.35,46.48 v22.54,46.67
  Bottom 0.406: v22.54,46.67 30.16,46.67 32.07,48.58 IC101.12
N$41  (via drill 0.3)
  Top 0.406: C103.2 28.57,41.27 27.18,42.67 Q101.1 27.3,43.31 v27.3,45.72
  Bottom 0.406: IC101.13 27.62,46.04 v27.3,45.72
N$42
  Top 0.406: Q102.2 22.35,29.72 20.95,31.11 C105.2
  Bottom 0.406: IC104.8 35.24,25.4 34.61,26.04 23.18,26.04 22.23,26.99 22.23,27.5 Q102.2
N$43
  Top 0.406: Q102.1 27.18,29.4 28.57,30.8 C106.2
  Bottom 0.406: IC104.7 37.78,26.35 37.47,26.67 28.13,26.67 Q102.1
O1
  Top 0.406: LED201.A 86.68,73.66 89.22,71.12 LED205.K
  Bottom 0.406: IC101.36 53.66,66.36 55.24,67.94 66.36,67.94 67.63,69.22 74.93,69.22 78.42,65.72 87.31,65.72 89.22,67.63 LED205.K
O2
  Top 0.406: LED202.A 86.68,53.34 89.22,50.8 LED206.K
  Bottom 0.406: IC101.35 53.66,63.82 55.24,65.41 60.96,65.41 63.5,62.87 69.22,62.87 77.15,54.93 83.82,54.93 LED202.A
O3  (via drill 0.3)
  Top 0.406: v59.69,62.55 v59.69,40.96 | LED203.A 86.68,33.66 89.22,31.11 LED207.K
  Bottom 0.406: IC101.34 53.66,61.28 54.93,62.55 v59.69,62.55 | v59.69,40.96 62.23,40.96 63.5,39.69 68.26,39.69 69.85,38.1 73.66,38.1 73.98,37.78 86.04,37.78 LED203.A
O4  (via drill 0.3)
  Top 0.406: v61.59,39.05 v61.59,57.47 | LED204.A 86.68,12.7 89.22,10.16 LED208.K | v63.18,16.83 v63.18,28.57
  Bottom 0.406: v61.59,57.47 60.01,59.05 54.61,59.05 53.98,58.42 49.21,58.42 IC101.33 | LED204.A 84.45,16.83 83.19,18.1 73.66,18.1 72.39,16.83 v63.18,16.83 | v61.59,39.05 61.59,38.42 63.18,36.83 66.04,36.83 67.63,35.24 67.63,29.53 66.67,28.57 v63.18,28.57
P10  (via drill 0.3)
  Top 0.406: v37.47,70.17 v37.47,43.5
  Bottom 0.406: X101.1 6.03,71.76 7.3,70.48 17.14,70.48 17.46,70.17 v37.47,70.17 | v37.47,43.5 IC101.14
P11  (via drill 0.3)
  Top 0.406: v35.56,67.63 35.56,41.27 35.24,40.96 IC101.15
  Bottom 0.406: X101.2 17.47,68.26 18.41,67.31 31.43,67.31 31.75,67.63 v35.56,67.63
P12  (via drill 0.3)
  Top 0.406: v14.61,40.01 14.61,44.45 13.65,45.4 v13.65,64.77
  Bottom 0.406: IC101.16 31.75,38.42 30.16,40.01 v14.61,40.01 | v13.65,64.77 X101.3
P13  (via drill 0.3)
  Top 0.406: v15.56,35.88 15.56,44.77 14.61,45.72 v14.61,61.28
  Bottom 0.406: IC101.17 v15.56,35.88 | v14.61,61.28 5.32,61.28 X101.4
P14  (via drill 0.3)
  Top 0.406: v17.46,34.29 17.46,45.4 16.51,46.35 v16.51,57.78
  Bottom 0.406: IC101.18 32.07,33.34 31.11,34.29 v17.46,34.29 | v16.51,57.78 5.33,57.78 X101.5
P15  (via drill 0.3)
  Top 0.406: v18.41,30.8 18.41,45.72 17.46,46.67 v17.46,54.29
  Bottom 0.406: IC101.19 v18.41,30.8 | v17.46,54.29 5.33,54.29 X101.6
P16  (via drill 0.3)
  Top 0.406: v19.37,28.89 19.37,46.04 18.41,46.99 v18.41,50.8
  Bottom 0.406: IC101.20 30.48,28.26 29.84,28.89 v19.37,28.89 | v18.41,50.8 5.34,50.8 X101.7
P17  (via drill 0.3)
  Top 0.406: v16.51,29.84 16.51,45.09 15.56,46.04 v15.56,47.31
  Bottom 0.406: IC101.21 36.83,28.26 35.56,29.53 31.11,29.53 30.8,29.84 v16.51,29.84 | v15.56,47.31 5.35,47.31 X101.8
PLUGGED  (via drill 0.3)
  Top 0.406: v10.16,72.71 10.16,85 CON101.3
  Bottom 0.406: IC101.39 36.83,73.98 35.56,72.71 v10.16,72.71
R1  (via drill 0.3)
  Top 0.406: v63.5,31.11 63.5,89.22 v63.18,89.53
  Bottom 0.406: IC101.22 54.29,30.8 54.61,31.11 v63.5,31.11 | v63.18,89.53 OK201.2
R2  (via drill 0.3)
  Top 0.406: v62.55,65.09 v62.55,51.12 | v44.13,49.85 v44.13,35.88
  Bottom 0.406: OK203.2 60.96,66.67 v62.55,65.09 | v62.55,51.12 51.44,51.12 50.16,49.85 v44.13,49.85 | v44.13,35.88 IC101.24
R3
  Top 0.406: IC101.26 53.66,40.96 56.52,43.81 OK205.2
R4  (via drill 0.3)
  Top 0.406: v46.99,46.04 46.99,25.08 46.67,24.77 v46.67,21.59
  Bottom 0.406: IC101.28 v46.99,46.04 | v46.67,21.59 54.29,21.59 54.93,20.95 OK207.2
SCK  (via drill 0.3)
  Top 0.406: IC104.13 v40.32,18.73 40.32,20.64 39.05,21.91 39.05,33.34 38.42,33.97 v38.42,58.74 | IC102.6 47.94,8.89 v46.99,9.84 46.67,10.16 v46.67,18.73
  Bottom 0.406: v38.42,58.74 IC101.8 | v46.67,18.73 v40.32,18.73 | SV101.3 25.72,11.43 29.21,11.43 30.8,9.84 v46.99,9.84
SPG
  Bottom 0.406: R107.2 R108.1 44.13,77.47 45.09,76.52 IC101.40
V+
  Top 0.813: X201.2 93.03,88.58 92.39,87.95 92.39,73.66 | 92.39,73.66 92.39,53.02 | 92.39,53.02 92.39,32.07 | 92.39,32.07 92.39,12.06 92.71,11.75 X205.2 | X204.2 92.39,32.07 | X203.2 92.71,52.7 92.39,53.02 | X202.2 92.71,73.34 92.39,73.66
V-NETZTEIL1
  Bottom 0.813: CON101.1 18.41,90.49 21.27,93.34 D103.A

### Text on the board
Bottom: bottom | MBCAN-Projekt | 20.07.2024 | (c) Dr.-Ing. Th. Wiesner | mbc92.brd
tNames: HW: 24.07.20 | AC | 0 | L | +18V | +18V | DC | Status | (c) Dr.-Ing. Th. Wiesner | MBCAN-Projekt | CH1 | CH2 | IN | CH3 | OUT | CH4 | mbc-92
bNames: 26.10.2019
